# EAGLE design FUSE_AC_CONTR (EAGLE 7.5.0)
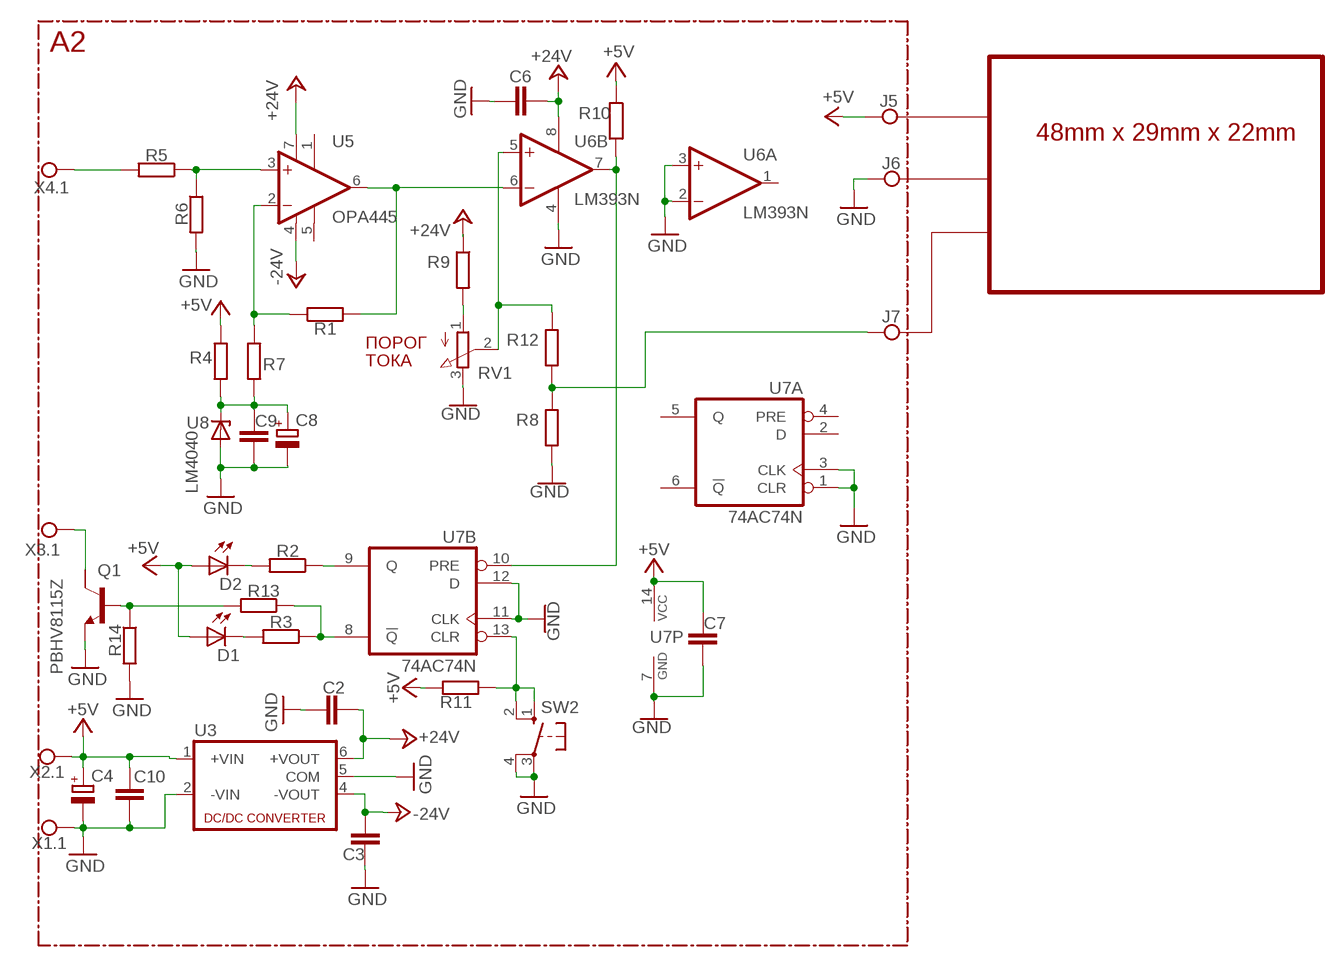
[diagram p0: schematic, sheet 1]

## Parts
C2  C-EUC0805  [C0805]
C3  C-EUC0805  [C0805]
C4  CPOL-EUE2.5-5  [E2,5-5]
C6  C-EUC0805  [C0805]
C7  C-EUC0805  [C0805]
C8  CPOL-EUE2.5-5  [E2,5-5]
C9  C-EUC0805  [C0805]
C10  C-EUC0805  [C0805]
D1  LED3MM  [LED3MM]
D2  LED3MM  [LED3MM]
J5  TPPAD1-20  [P1-20]
J6  TPPAD1-20  [P1-20]
J7  TPPAD1-20  [P1-20]
Q1  PBHV8115Z  [SOT223]
R1  R-EU_R0805  [R0805]
R2  R-EU_R0805  [R0805]
R3  R-EU_R0805  [R0805]
R4  R-EU_R0805  [R0805]
R5  R-EU_R0805  [R0805]
R6  R-EU_R0805  [R0805]
R7  R-EU_R0805  [R0805]
R8  R-EU_R0805  [R0805]
R9  R-EU_R0805  [R0805]
R10  R-EU_R0805  [R0805]
R11  R-EU_R0805  [R0805]
R12  R-EU_R0805  [R0805]
R13  R-EU_R0805  [R0805]
R14  R-EU_R0805  [R0805]
RV1  PTV09A  PV09A  [PTV09]
SW2  SPST Push Button  10-XX  [B3F-10XX]
U3  NMA  [NMA]
U5  OPA445  OPA131P  [DIL08]
U6  LM393N  [DIL08]
U7  74AC74N  [DIL14]
U8  LM4040  [SOT23]
X1.1  TPPAD1-20  [P1-20]
X2.1  TPPAD1-20  [P1-20]
X3.1  TPPAD1-20  [P1-20]
X4.1  TPPAD1-20  [P1-20]

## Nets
+5V: C4.+ C7.1 C10.2 D1.A D2.A J5.TP R4.1 R10.1 R11.1 U3.1(+VIN) U7.14(P:VCC) X2.1.TP
+24V: C2.2 C6.1 R9.1 U3.6(+VOUT) U5.7(V+) U6.8(P:V+)
-24V: C3.2 U3.4(-VOUT) U5.4(V-)
GND: C2.1 C3.1 C4.- C6.2 C7.2 C8.- C9.2 C10.1 J6.TP Q1.3(E) R6.2 R8.2 R14.2 RV1.3(E) SW2.3(P) SW2.4(P1) U3.2(-VIN) U3.5(COM) U6.2(A:-IN) U6.3(A:+IN) U6.4(P:V-) U7.1(A:CLR) U7.3(A:CLK) U7.7(P:GND) U7.11(B:CLK) U7.12(B:D) U8.2(A) X1.1.TP
N$3: R5.1 R6.1 U5.3(+IN)
N$4: R1.1 R7.1 U5.2(-IN)
N$5: R1.2 U5.6(OUT) U6.6(B:-IN)
N$6: C8.+ C9.1 R4.2 R7.2 U8.1(C)
N$7: R9.2 RV1.1(A)
N$8: R12.1 RV1.2(S) U6.5(B:+IN)
N$9: R11.2 SW2.1(S) SW2.2(S1) U7.13(B:CLR)
N$10: D2.K(C) R2.2
N$11: R3.1 R13.1 U7.8(B:!Q)
N$12: J7.TP R8.1 R12.2
N$13: R2.1 U7.9(B:Q)
N$14: D1.K(C) R3.2
N$17: Q1.1(B) R13.2 R14.1
N$21: Q1.2(C) X3.1.TP
N$23: R5.2 X4.1.TP
N$42: R10.2 U6.7(B:OUT) U7.10(B:PRE)
Unconnected: Q1.4(C) U5.1(TRIM1) U5.5(TRIM2) U6.1(A:OUT) U7.2(A:D) U7.4(A:PRE) U7.5(A:Q) U7.6(A:!Q)

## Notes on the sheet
- А2
- 48mm x 29mm x 22mm
- ПОРОГ
- ТОКА

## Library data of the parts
C2 C3 C6 C7 C9 C10 = rcl:C-EU: CAPACITOR, European symbol
C4 C8 = rcl:CPOL-EU: POLARIZED CAPACITOR, European symbol
D1 D2 = led:LED: LED
J5-J7 X1.1 X2.1 X3.1 X4.1 = testpad:TP: Test pad
Q1 = transistor-npn:PBHV8115Z
R1-R14 = rcl:R-EU_: RESISTOR, European symbol
RV1 = pot:PV09A
SW2 = switch-omron:10-XX: OMRON SWITCH; MPN: B3F-1000; OC_FARNELL: 176432; OC_NEWARK: 36M3542
U3 = dc-dc-converter:NMA: DC-DC CONVERTER; MF: C & D TECHNOLOGIES, INC; MPN: NMA0515SC; OC_FARNELL: 1021434; OC_NEWARK: 61K3064
U5 = burr-brown:OPA131: Operational Amplifiers General Purpose FET-Input; OC_FARNELL: unknown; OC_NEWARK: unknown
U6 = linear:LM393: COMPARATOR
U7 = 74xx-eu:74*74: Dual D type positive edge triggered FLIP FLOP, preset and clear
U8 = diode:LM4040: PrecisionMicropowerShuntVoltageReference

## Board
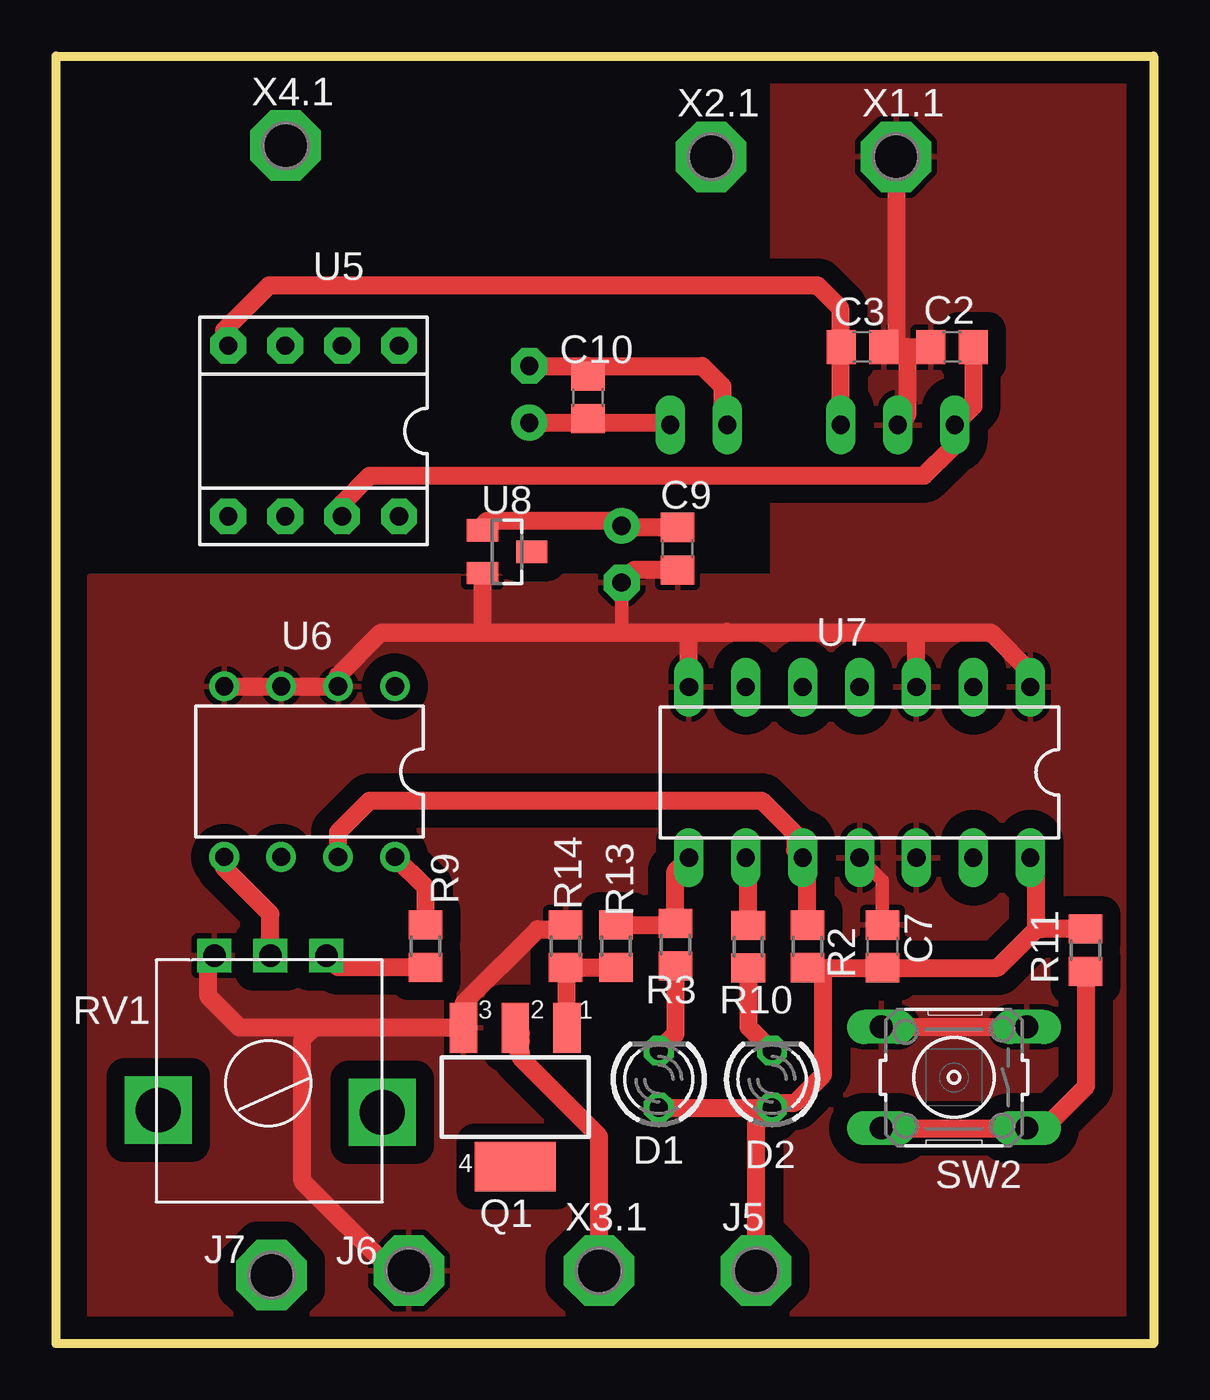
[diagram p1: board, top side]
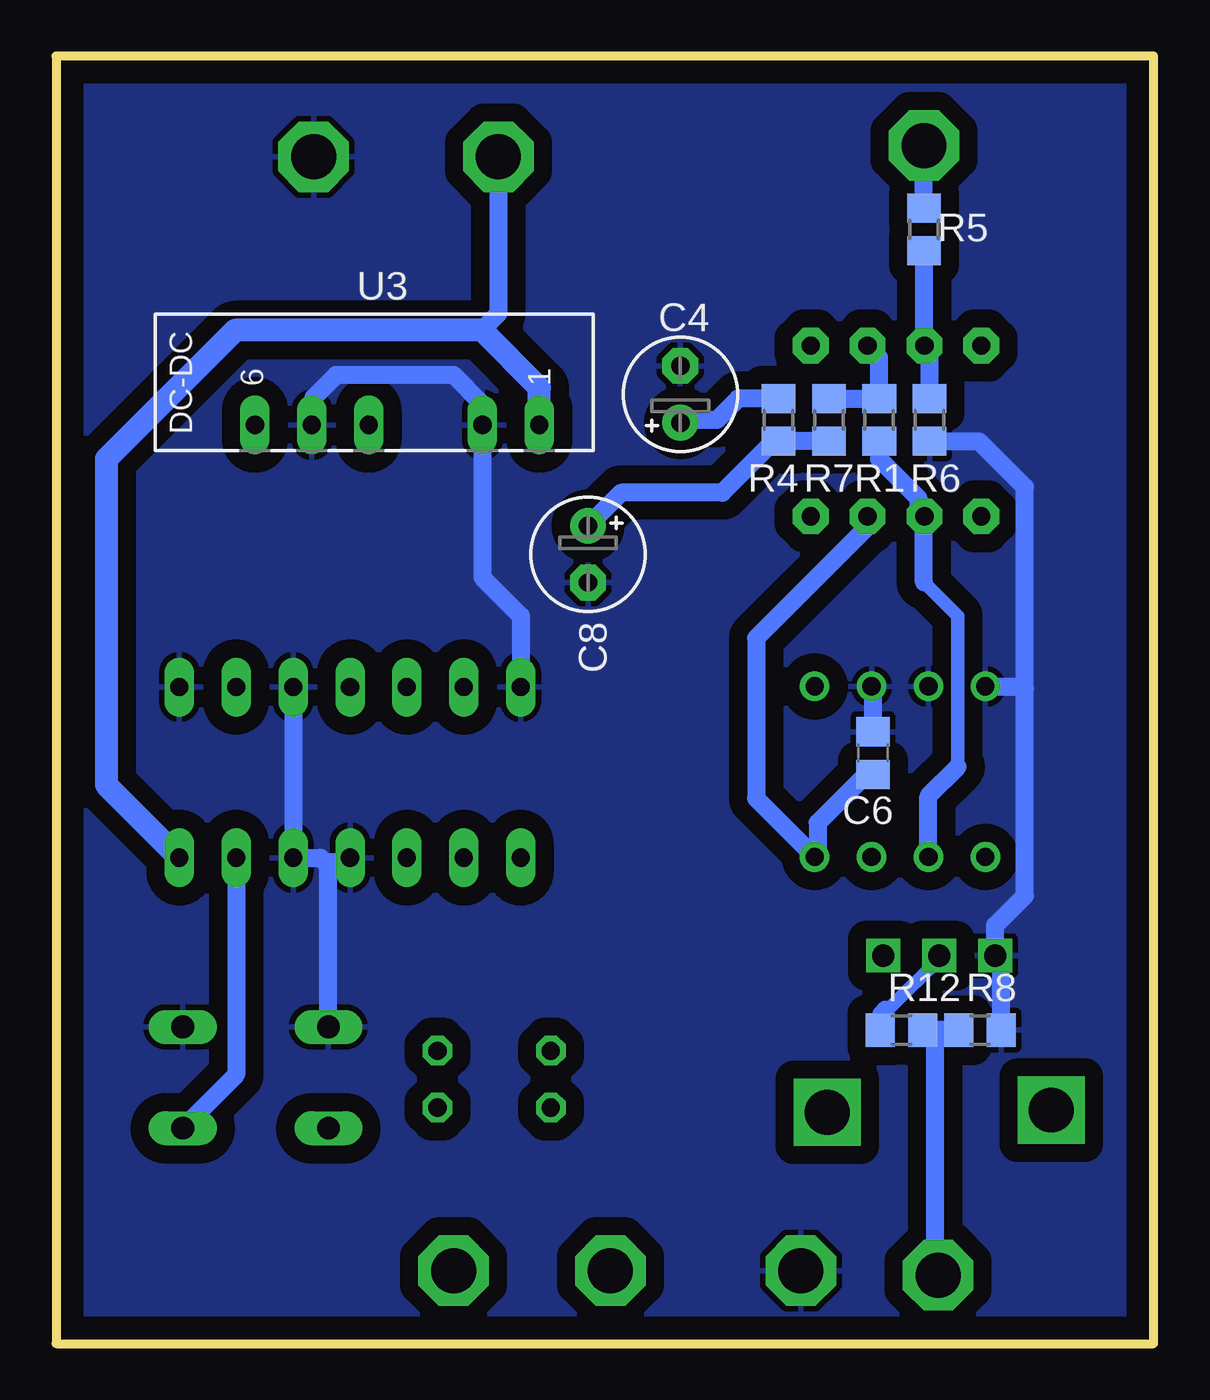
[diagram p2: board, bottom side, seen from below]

Size 49 x 57.5 mm. Coordinates in mm from the lower left corner, seen from the top.
Outline: 0,0 0,57.5 49,57.5 49,0 0,0
Copper layers (1*16): Top 0.035mm / dielectric 1.5mm / Bottom 0.035mm
Design rules "default": minimum track width 10mil, minimum drill 24mil, track to track 8mil, track to pad 8mil, pad to pad 8mil, via to via 8mil, smd to smd 8mil, copper to edge 40mil, drill to drill 8mil, minimum pad ring 10mil, minimum via ring 8mil, stop-mask expansion 4mil, vias tented up to drill 0mil, thermal gap 10mil

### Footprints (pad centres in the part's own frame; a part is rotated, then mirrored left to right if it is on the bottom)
C0805 = smd 1.3 x 1.5: 1 -0.95,0; 2 0.95,0
E2,5-5 = drill 0.813 pad 1.6: + -1.27,0 | drill 0.813 pad 1.6 octagon: - 1.27,0
LED3MM = drill 0.813 octagon: A -1.27,0; K 1.27,0
P1-20 = drill 2.007 pad 3.15 octagon: TP 0,0
SOT223 = smd 1.219 x 2.235: 1 -2.311,-3.099; 2 0,-3.099; 3 2.311,-3.099 | smd 3.6 x 2.2: 4 0,3.099
R0805 = smd 1.3 x 1.5: 1 -0.95,0; 2 0.95,0
PTV09 = drill 1 square: 1 -2.5,0; 2 0,0; 3 2.5,0 | drill 2 square: P$4 -5,7; P$5 5,6.9
B3F-10XX = drill 1.016 long: 1 -3.251,2.261; 2 3.251,2.261; 3 -3.251,-2.261; 4 3.251,-2.261
NMA = drill 0.813 long: 1 0,6.35; 2 0,3.81; 4 0,-1.27; 5 0,-3.81; 6 0,-6.35
DIL08 = drill 0.813 pad 1.6 octagon: 1 -3.81,-3.81; 2 -1.27,-3.81; 3 1.27,-3.81; 4 3.81,-3.81; 5 3.81,3.81; 6 1.27,3.81; 7 -1.27,3.81; 8 -3.81,3.81
DIL08' = drill 0.813 pad 1.27: 1 -3.81,-3.81; 2 -1.27,-3.81; 3 1.27,-3.81; 4 3.81,-3.81; 5 3.81,3.81; 6 1.27,3.81; 7 -1.27,3.81; 8 -3.81,3.81
DIL14 = drill 0.813 long: 1 -7.62,-3.81; 2 -5.08,-3.81; 3 -2.54,-3.81; 4 0,-3.81; 5 2.54,-3.81; 6 5.08,-3.81; 7 7.62,-3.81; 8 7.62,3.81; 9 5.08,3.81; 10 2.54,3.81; 11 0,3.81; 12 -2.54,3.81; 13 -5.08,3.81; 14 -7.62,3.81
SOT23 = smd 1 x 1.4: 1 -0.95,-1.1; 2 0.95,-1.1; 3 0,1.1

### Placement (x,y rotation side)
C2  40,44.5 0 top
C3  36,44.5 180 top
C4  21.12,42.39 90 bottom
C6  12.52,26.37 90 bottom
C7  36.9,17.73 90 top
C8  25.25,35.25 270 bottom
C9  27.75,35.5 270 top
C10  23.75,42.25 270 top
D1  26.91,11.8 90 top
D2  31.96,11.8 90 top
J5  31.25,3.25 0 top
J6  15.75,3.25 0 top
J7  9.62,3.05 0 top
Q1  20.5,11 180 top
R1  12.25,41.25 270 bottom
R2  30.91,17.73 270 top
R3  27.66,17.81 270 top
R4  16.75,41.25 270 bottom
R5  10.25,49.75 90 bottom
R6  10,41.25 270 bottom
R7  14.5,41.25 270 bottom
R8  7.75,14 0 bottom
R9  16.5,17.75 270 top
R10  33.55,17.73 90 top
R11  45.96,17.56 270 top
R12  11.25,14 0 bottom
R13  25,17.75 270 top
R14  22.75,17.75 90 top
RV1  9.57,17.32 180 top
SW2  40.09,11.88 180 top
U3  33.77,41.02 270 bottom
U5  11.5,40.75 180 top
U6  LM393N  [DIL08']  11.32,25.54 180 top
U7  35.88,25.5 180 top
U8  20.14,35.36 270 top
X1.1  37.5,53 0 top
X2.1  29.25,53 0 top
X3.1  24.25,3.25 0 top
X4.1  10.25,53.5 0 top

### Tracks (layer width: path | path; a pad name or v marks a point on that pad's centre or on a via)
+5V
  Top 0.813: D1.A D2.A | D2.A 32.18,10.75 33,10.75 34.25,12 34.25,16.54 34.5,16.79 | R10.1 34.5,16.79 | 34.5,16.79 C7.1 42.03,16.79 43.75,18.5 43.75,18.75 | C4.+ 23.5,41.12 | 23.5,41.12 27.32,41.12 U3.1 | C10.2 23.68,41.3 23.5,41.12 | J5.TP 31.25,9.82 D2.A | 43.75,18.75 43.75,21.44 U7.14 | R11.1 43.99,18.51 43.75,18.75
  Bottom 0.813: X2.1.TP 29.25,46 30,45.25 | R4.1 18.55,42.2 19.5,41.25 21,41.25 C4.+
  Bottom 1.016: U3.1 27.42,42.67 30,45.25 41,45.25 46.75,39.5 46.75,24.95 U7.14
+24V
  Top 0.813: R9.1 16.5,20.36 U6.8 | U5.7 12.77,37.52 14,38.75 38.75,38.75 40,40 40,40.91 U3.6 40.95,41.85 C2.2
  Bottom 0.813: C6.1 12.83,25.42 15,23.25 15,21.86 U6.8 17.75,24.35 17.75,31.5 12.77,36.48 U5.7
-24V
  Top 0.813: U3.4 C3.2 35,44.55 35,46.25 34,47.25 9.5,47.25 7.5,45.25 7.5,44.75 U5.4
GND
  Top 0.61: C8.- 25.25,31.75 | C7.2 36.9,20.68 U7.11
  Top 0.813: U6.4 U6.3 U6.2 12.59,29.84 14.5,31.75 19,31.75 | 19,31.75 25.25,31.75 28.5,31.75 | 28.5,31.75 30,31.75 | 30,31.75 38.25,31.75 | 38.25,31.75 41.75,31.75 43.5,30 U7.1 | U7.3 38.41,31.59 38.25,31.75 | U7.7 28.25,31.5 28.5,31.75 | 29.96,31.79 30,31.75 | C9.2 25.82,34.55 C8.- | C4.- 23.75,43.66 | 23.75,43.66 28.84,43.66 29.75,42.75 29.75,41.23 U3.2 | C10.1 23.75,43.66 | SW2.4 SW2.3 | 38,44.5 C2.1 | C3.1 38,44.5 | 38,44.5 38,44 | 38,44 38,41.45 U3.5 | X1.1.TP 37.5,44.5 38,44 | U8.2 19.04,31.79 19,31.75 | 11.5,14.1 Q1.3 18.19,15.19 21.5,18.5 22.3,18.5 R14.2 | 11.5,14.1 8.2,14.1 6.8,15.5 6.8,17.05 RV1.3 | J6.TP 15,3.25 11,7.25 11,13.6 11.5,14.1
  Bottom 0.813: SW2.4 36.84,21.34 37,21.5 | 37,21.5 36.07,21.5 U7.11 | 37,21.5 37.2,21.7 U7.12 U7.3 | R8.2 6.8,17.05 RV1.3 7.07,18.68 5.75,20 5.75,29.25 | U7.7 28.25,32.5 29.96,34.21 U3.2 29.96,41.96 31.25,43.25 36.5,43.25 37.5,42.25 37.5,41.1 U3.5 | R6.2 7.8,40.3 5.75,38.25 5.75,29.25 | U6.4 5.85,29.35 5.75,29.25 | C6.2 12.52,29.28 U6.2
  pour Bottom (isolate 0.813): 0.5,56.75 48.25,56.75 48.25,1 0.5,1
  pour Top (isolate 0.813): 6,34.25 41.5,34.25 46.25,29.5 47.75,28 47.75,1 1.5,1 1.5,34.25
  pour Top (isolate 0.813): 33,56.25 47.75,56.25 47.75,28.25 32,28.25 32,56.25
N$3
  Bottom 0.813: R5.1 10.23,48.78 U5.3 10,44.33 R6.1
N$4
  Bottom 0.813: U5.2 12.25,44.04 R1.1 R7.1
N$5
  Bottom 0.61: 8.75,25.75 8.75,32.5 10.25,34
  Bottom 0.813: U6.6 10.05,24.45 8.75,25.75 | 10.25,34 10.25,36.92 U5.6 10.5,37.21 10.5,37.75 12.25,39.5 R1.2
N$6
  Top 0.813: C9.1 25.32,36.45 C8.+ 25.02,36.75 19.25,36.75 19.04,36.54 U8.1
  Bottom 0.813: R7.2 R4.2 16.95,40.3 19.25,38 23.77,38 C8.+
N$7
  Top 0.813: R9.2 12.6,16.8 RV1.1
  Bottom 0.813: 12.2,17.2 RV1.1
N$8
  Top 0.813: RV1.2 9.57,19.18 7.5,21.25 U6.5
  Bottom 0.61: RV1.2 9.57,17.18 11.75,15 12,15 12.25,14.75 12.25,14.05 R12.1
N$9
  Top 0.813: SW2.2 SW2.1 43.46,9.5 44,9.5 45.96,11.46 R11.2
  Bottom 0.813: U7.13 40.95,12.01 SW2.1
N$10
  Top 0.813: R2.2 30.91,14.13 D2.K
N$11
  Top 0.813: U7.8 27.66,21.09 R3.1 27.59,18.7 R13.1
N$12
  Bottom 0.813: R8.1 9.75,14 | 9.75,14 R12.2 | J7.TP 9.75,3.05 9.75,14
N$13
  Top 0.813: R2.1 30.91,21.59 U7.9
N$14
  Top 0.813: R3.2 27.66,13.82 D1.K
N$17
  Top 0.813: Q1.1 22.81,16.74 R14.1 R13.2
N$21
  Top 0.813: X3.1.TP 24.25,9.25 20.75,12.75 20.75,13 20.5,13.25 20.75,13.5 20.75,13.85 Q1.2
N$23
  Bottom 0.813: R5.2 X4.1.TP
N$42
  Top 0.813: R10.2 33.55,21.48 U7.10 33,22.03 33,22.75 31.5,24.25 14,24.25 12.59,22.84 U6.7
